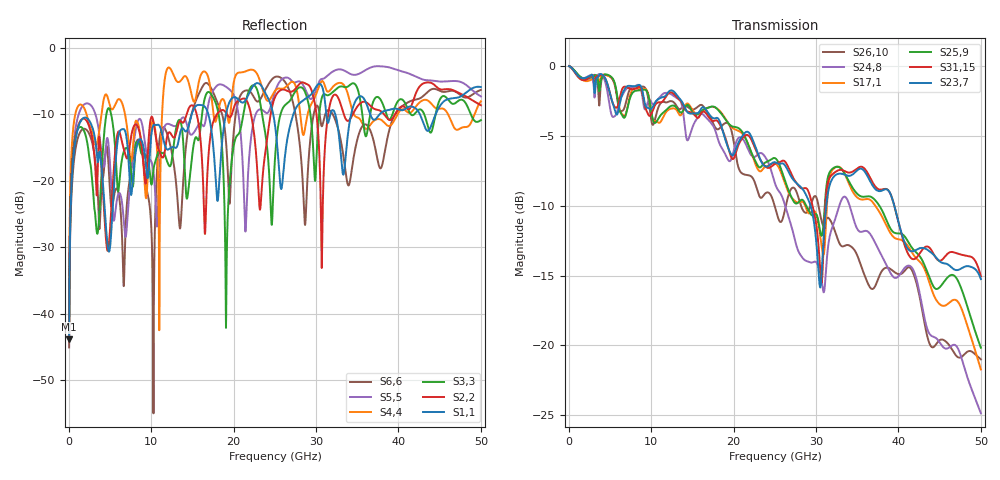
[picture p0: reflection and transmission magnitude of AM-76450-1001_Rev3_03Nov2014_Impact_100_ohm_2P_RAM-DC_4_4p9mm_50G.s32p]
! IMPORTANT NOTE: This model should not be used to evaluate
! electrical signals with a greater than 50 GHz. of frequency content.
! Please apply appropriate analysis techniques when reviewing the results of
! your simulations.
!  COPYRIGHT 2008, BY MOLEX INCORPORATED
!  ALL INTERNATIONAL RIGHTS RESERVED
!  THIS FILE CONTAINS MOLEX INCORPORATED CONFIDENTIAL INFORMATION
! >>>>>>>>>>>>>>>>  USER AGREEMENT  <<<<<<<<<<<<<<<<<<<
! The information on this media is the property of MOLEX Incorporated
! and  has been provided to you free of charge. Molex does not
! guarantee that the information is error-free, nor does MOLEX  make
! any representations, warranty or guarantee that the information is
! accurate, correct, reliable or up-to-date. MOLEX expressly
! disclaims all implied warranties regarding this information,
! including but not limited to any implied  warranties of
! merchantability or fitness for a particular purpose. MOLEX does
! not warrant that the media will work correctly in your multi- user
! or network environment.
! MOLEX will in no case be liable for your use, or the results of
! your use, of the software and other information contained on this
! media or  any accompanying written materials.  IT IS YOUR
! RESPONSIBILITY TO VERIFY THE RESULTS OF YOUR USE OF THIS
! INFORMATION IN YOUR OWN PARTICULAR ENGINEERING AND PRODUCT
! ENVIRONMENT, AND YOU ASSUME THE ENTIRE RISK OF DOING SO OR
! FAILING TO DO SO.  In no event will MOLEX be liable for any
! direct, indirect, incidental or consequential damages arising from
! your use of, or your inability to use, software, product simulations
! and other information contained on this media or any accompanying
! written materials.
! This model has not been validated with empirical data.
! This model was solved using HFSS.  TDR results can run 5-8 ohms low
! Touchstone file from project AM-76450-1001_Rev3_03Nov2014_Impact_100_ohm_2P_RAM-DC_4_4p9mm_50G
! Exported from HFSS 15.0.0
! Terminal data exported
! Port[1] = B1_T1
! Port[2] = C1_T1
! Port[3] = E1_T1
! Port[4] = F1_T1
! Port[5] = A2_T1
! Port[6] = B2_T1
! Port[7] = D2_T1
! Port[8] = E2_T1
! Port[9] = B3_T1
! Port[10] = C3_T1
! Port[11] = E3_T1
! Port[12] = F3_T1
! Port[13] = A4_T1
! Port[14] = B4_T1
! Port[15] = D4_T1
! Port[16] = E4_T1
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# GHZ S MA R 50.000000
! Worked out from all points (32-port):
!   2500 points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, 20 MHz to 50 GHz, reference 50 ohm
!   strongest paths, dB at 20 MHz, 12.52 GHz, 25.02 GHz, 37.52 GHz, 50 GHz:
!     S23,7: 0.0, -1.7, -6.9, -8.9, -15.3
!     S31,15: 0.0, -1.9, -7.0, -8.8, -15.0
!     S25,9: 0.0, -2.8, -6.6, -9.9, -20.2
!     S17,1: 0.0, -3.0, -7.0, -10.3, -21.7
!     S24,8: 0.0, -2.1, -8.4, -13.1, -24.9
!     S26,10: 0.0, -2.5, -10.1, -15.3, -21.0
!   lowest |S11| = -43.8 dB at 20 MHz (marker M1), VSWR 1.01, Z = 50 + j0.644 ohm
!   |S11| at or under -10 dB: start of sweep to 14.9 GHz; 16.91 GHz to 19.06 GHz (2.149 GHz wide, 11.9 % of centre); 24.79 GHz to 27.25 GHz (2.459 GHz wide, 9.45 % of centre)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
